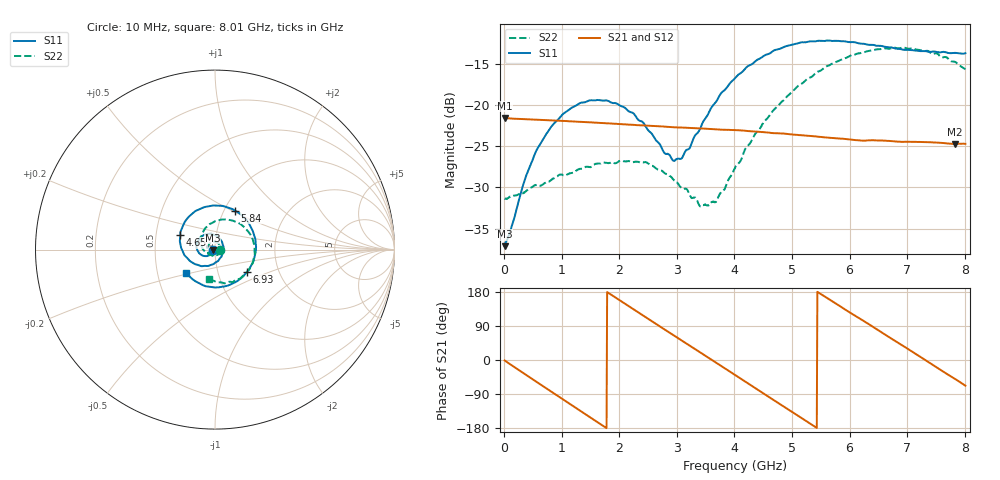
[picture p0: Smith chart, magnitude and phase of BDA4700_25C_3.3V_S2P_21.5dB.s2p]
!Agilent Technologies,E5071B,MY42404982,A.09.10
!Date: Mon Oct 20 18:12:05 2025
!Data & Calibration Information:
!Freq	S11:SOLT2(ON)	S21:SOLT2(ON)	S12:SOLT2(ON)	S22:SOLT2(ON)
# Hz S RI R 50
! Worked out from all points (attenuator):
!   801 points, 10 MHz to 8.01 GHz, reference 50 ohm
!   highest |S21| = -21.58 dB at 10 MHz (marker M1); lowest = -24.7 dB at 7.83 GHz (marker M2)
!   lowest |S11| = -37.1 dB at 10 MHz (marker M3), VSWR 1.03, Z = 48.6 - j0.137 ohm
!   |S11| at or under -10 dB: start of sweep to end of sweep
!   |S22| runs from -32.3 to -13.0 dB; largest |S21 - S12| = 0.00095
!   S11 on the Smith chart (normalised r, x): 10 MHz: 0.97, -0.00; 4.65 GHz: 0.67, +0.12; 5.84 GHz: 1.12, +0.52; 6.93 GHz: 1.38, -0.36; 8.01 GHz: 0.70, -0.19
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1e7  -0.0138 -0.00141  0.0834 -0.0018  0.0833 -0.00185  0.027 -0.000801
3.7e8  -0.0246 -0.0262  0.0647 -0.0506  0.0646 -0.0506  0.0223 -0.0197
5.8e8  -0.0412 -0.0356  0.0415 -0.0701  0.0416 -0.07  0.0145 -0.0292
1e9  -0.0828 -0.0246  -0.0162 -0.0785  -0.0162 -0.0786  -0.0148 -0.0349
1.35e9  -0.1029 0.0123  -0.0576 -0.0541  -0.0577 -0.0541  -0.0369 -0.0181
1.77e9  -0.0835 0.0667  -0.0776 -0.00164  -0.0775 -0.00163  -0.0427 0.0131
2.07e9  -0.0442 0.0869  -0.0671 0.0366  -0.0672 0.0367  -0.0305 0.034
2.68e9  0.0379 0.0454  -0.00146 0.0743  -0.0016 0.0743  0.0138 0.038
2.93e9  0.046 0.0036  0.0292 0.0674  0.0291 0.0672  0.0256 0.0246
3.06e9  0.0428 -0.0196  0.0433 0.0589  0.0427 0.0592  0.0284 0.0145
3.43e9  -0.00181 -0.0757  0.0687 0.0218  0.0688 0.0219  0.0199 -0.0138
3.69e9  -0.0544 -0.0908  0.0705 -0.0097  0.0706 -0.00994  0.000888 -0.0261
4.01e9  -0.1269 -0.0717  0.0544 -0.0447  0.0545 -0.0446  -0.032 -0.0263
4.65e9  -0.1935 0.0828  -0.0148 -0.066  -0.0146 -0.0662  -0.0796 0.043
5.35e9  -0.0529 0.238  -0.064 -0.00978  -0.064 -0.0102  -0.0156 0.1484
5.84e9  0.1118 0.2174  -0.0489 0.0391  -0.0487 0.0392  0.0943 0.1625
6.26e9  0.2092 0.1071  -0.0123 0.0595  -0.0115 0.0596  0.1831 0.1026
6.68e9  0.2201 -0.0433  0.0295 0.0529  0.0296 0.0528  0.2205 -0.00205
6.93e9  0.1787 -0.1232  0.0477 0.0361  0.0479 0.0358  0.2121 -0.0716
7.42e9  0.0248 -0.2093  0.0584 -0.0109  0.0584 -0.0109  0.1207 -0.166
7.83e9  -0.1151 -0.1731  0.0374 -0.0445  0.0373 -0.0446  0.0112 -0.1824
8.01e9  -0.1607 -0.1297  0.022 -0.0539  0.0223 -0.0538  -0.0321 -0.1617
